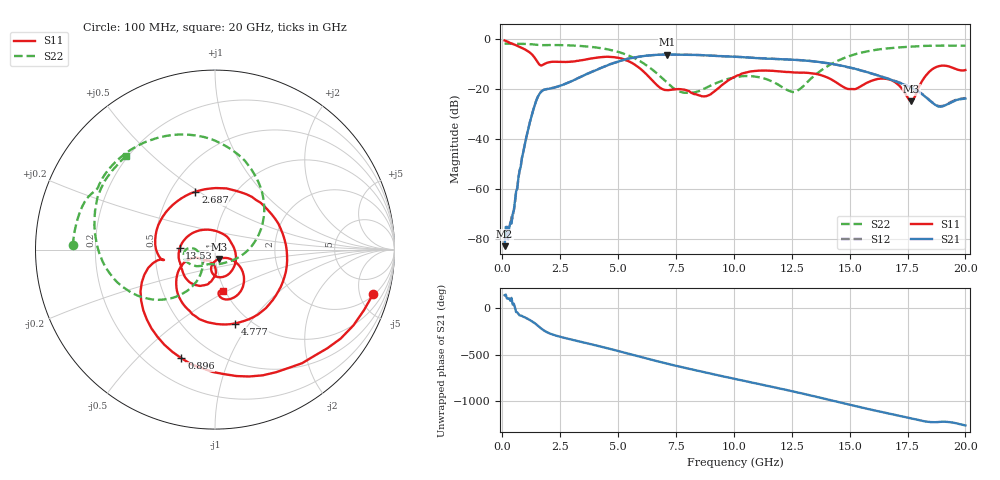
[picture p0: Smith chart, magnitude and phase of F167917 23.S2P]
!  2-Port S-parameters saved by WinCal
! VAR MeasName=S-Parameters (CALIBRATED_DATA) read from VNA (N5242A)
! VAR MeasDate=2016-11-22 9:00:50
! VAR NAME=F167917 23
! VAR FILENAME=F167917 23.S2P
! VAR DATE=2016-11-22 9:00:50
! VAR PHYS_PORTS=1,2
# Hz S DB R 50
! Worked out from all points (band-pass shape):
!   401 points, 100 MHz to 20 GHz, reference 50 ohm
!   highest |S21| = -6.39 dB at 7.115 GHz (marker M1); lowest = -83.0 dB at 100 MHz (marker M2)
!   |S21| within 3 dB of the highest: 4.953 GHz to 13.7 GHz (8.745 GHz wide, 93.8 % of centre)
!   lowest |S11| = -25.0 dB at 17.66 GHz (marker M3), VSWR 1.12, Z = 51.9 - j5.42 ohm
!   |S11| at or under -10 dB: 1.566 GHz to 1.855 GHz (288.6 MHz wide, 16.9 % of centre); 5.65 GHz to end of sweep
!   |S22| runs from -21.7 to -2.0 dB; largest |S21 - S12| = 0.0046
!   S11 on the Smith chart (normalised r, x): 100 MHz: 2.17, -6.63; 896 MHz: 0.34, -0.68; 2.687 GHz: 0.66, +0.48; 4.777 GHz: 0.85, -0.86; 13.53 GHz: 0.67, +0.01; 20 GHz: 0.98, -0.48
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1e8  -0.76 -15.5  -82.97 139.8  -82.44 -101.7  -2.02 178.3
3.4875e8  -1.82 -46.7  -73.41 80.0  -74.34 66.0  -2.05 174.2
8.96e8  -3.97 -107.2  -45.81 -89.5  -45.69 -89.5  -2.14 165.1
1.5925e9  -10.31 -169.7  -22.33 160.6  -22.28 160.5  -2.58 153.8
2.687e9  -9.36 108.8  -18.22 41.6  -18.20 41.3  -2.66 136.2
3.43325e9  -8.67 35.9  -15.11 -2.3  -15.11 -2.3  -3.01 120.3
4.03025e9  -7.67 -17.2  -12.61 -37.7  -12.61 -37.6  -3.54 105.4
4.7765e9  -7.40 -74.9  -9.89 -84.0  -9.85 -84.0  -4.78 83.3
5.62225e9  -9.85 -130.1  -7.74 -139.2  -7.70 -139.4  -7.47 52.6
6.7665e9  -19.30 -154.7  -6.47 147.1  -6.47 147.0  -14.65 -0.5
7.11475e9  -20.60 -140.3  -6.39 125.7  -6.41 125.6  -17.58 -21.2
8.7565e9  -23.06 -111.6  -6.70 31.4  -6.69 31.4  -19.87 -121.7
1.005e10  -15.24 -95.9  -7.28 -38.2  -7.27 -38.1  -15.56 -154.1
1.1443e10  -12.82 -132.2  -8.05 -111.9  -7.96 -111.9  -16.34 177.7
1.258725e10  -13.55 -154.4  -8.48 -173.6  -8.47 -173.9  -21.35 -153.9
1.338325e10  -13.90 -176.0  -9.04 140.5  -9.04 140.4  -15.56 -120.1
1.35325e10  -14.09 178.0  -9.22 131.9  -9.21 131.6  -14.41 -119.7
1.517425e10  -20.24 33.0  -11.89 35.4  -11.95 35.7  -6.46 -145.7
1.67165e10  -16.37 -85.7  -16.21 -51.3  -16.19 -50.6  -3.86 -177.2
1.766175e10  -25.00 -68.0  -19.62 -103.8  -19.51 -103.1  -3.22 166.8
1.865675e10  -11.75 -53.0  -26.22 -142.5  -26.10 -141.8  -2.84 151.1
2e10  -12.60 -78.6  -23.95 -177.4  -23.79 -177.2  -2.86 133.3
